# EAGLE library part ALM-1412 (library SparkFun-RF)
GPS Antenna Amp Filter and Amp built into one. Very small package.
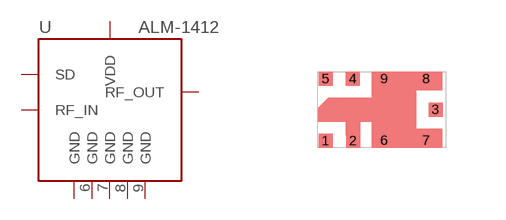
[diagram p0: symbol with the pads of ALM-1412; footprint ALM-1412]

Designator prefix -

## ALM-1412SMD  [ALM-1412]
1  SD
2  GND
3  RF_OUT
4  VDD
5  RF_IN
6  GND
7  GND
8  GND
9  GND

## Footprint ALM-1412 (pad centres in mm)
smd 0.35 x 0.35: 1 0,0.17; 2 0.69,0.17; 3 2.75,0.95; 4 0.68,1.72; 5 0,1.72; 6 1.47,0.18; 7 2.52,0.18; 8 2.52,1.72; 9 1.47,1.72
